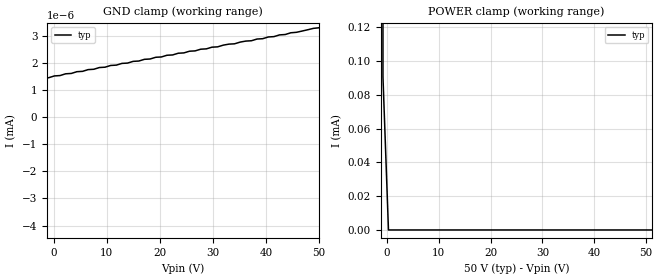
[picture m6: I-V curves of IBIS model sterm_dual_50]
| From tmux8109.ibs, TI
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| sterm_dual_50
[Model]   sterm_dual_50
Model_type   Terminator
|   typ   min   max
C_comp   2.533030e-12   NA   NA
[Voltage Range]   50   NA   NA
[Temperature Range]   27   NA   NA
[Power Clamp Reference]   50   NA   NA
[GND Clamp Reference]   0   NA   NA
[GND Clamp]
|   Voltage   I(typ)   I(min)   I(max)
-55V      -1.133A    NA         NA
-50.76V   -890uA     NA         NA
-49.7V    -653.5pA   NA         NA
-44.39V   -458.1pA   NA         NA
-30.61V   260.2pA    NA         NA
-13.64V   991.4pA    NA         NA
6.515V    1.753nA    NA         NA
33.03V    2.692nA    NA         NA
34.09V    2.704nA    NA         NA
36.21V    2.805nA    NA         NA
37.27V    2.817nA    NA         NA
50V       3.296nA    NA         NA
[POWER Clamp]
|   Voltage   I(typ)   I(min)   I(max)
-5V       744mA      NA         NA
-1.818V   145.4mA    NA         NA
-757.6mV  90.5uA     NA         NA
303mV     3.293nA    NA         NA
100V      -690.1pA   NA         NA
